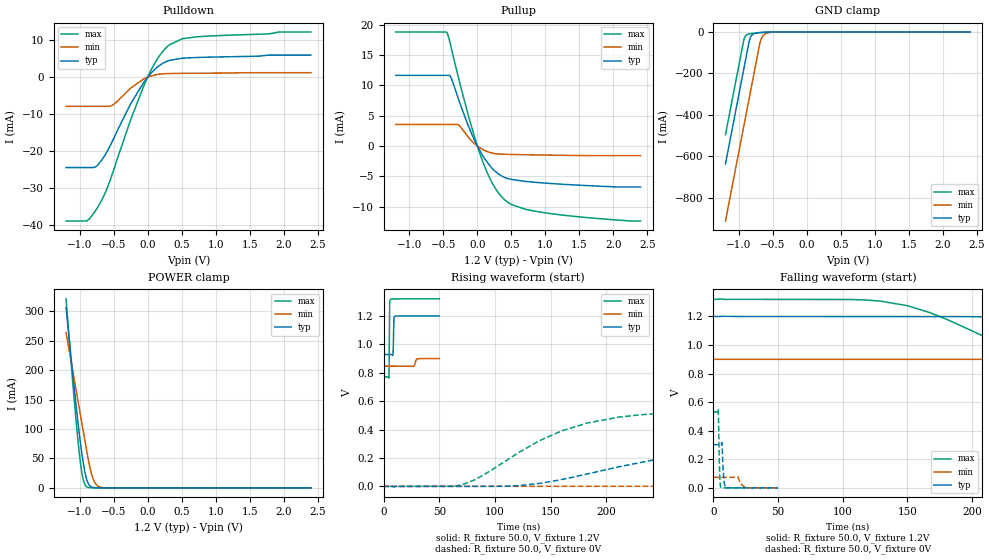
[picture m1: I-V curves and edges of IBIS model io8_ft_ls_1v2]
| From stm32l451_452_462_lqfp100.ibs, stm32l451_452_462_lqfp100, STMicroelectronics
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[Model]   io8_ft_ls_1v2
Model_type I/O
Polarity   Non-Inverting
Enable   Active-Low
| CAP_THRESHOLD on pad IOFT is "UDTCAPC" :
| Rising=30.00f vddiom   Falling=70.00f vddiom
| C_comp min and max val. don't necessarily correlate with the min and max pvt
| but are the smallest and greatest pad capacitance found.
| var   typ   min   max
C_comp   1.83455pF  1.76050pF  1.83491pF
|C_comp_pullup   1.06365pF  1.01770pF  1.04720pF
|C_comp_pulldown   770.90000fF  742.80001fF  787.71000fF
Vinl = 270.0mV
Vinh = 924.0mV
Vmeas = 600.0mV   | Reference voltage for timing measurements
Cref  = 50.0pF   | Timing specification test load capacitance value
Rref  = 100.0MOhm   | Timing specification test load resistance value
Vref  = 600.0mV   | Timing specification test load voltage
[Model Spec]
| TIME_THRESHOLD on pin ZIV12 is "CMOS" :
| Rising=50.00f vdd   Falling=50.00f vdd
Vinl 458.70000mV 364.70000mV 499.70000mV
Vinh 728.30000mV 548.30000mV 792.30000mV
| variable   typ   min   max
[Temperature Range] 25.0 140.0 -40.0
| variable   typ   min   max
[Voltage Range] 1.2V 900.0mV 1.32V
| variable   typ   min   max
[POWER Clamp Reference] 1.2V 900.0mV 1.32V
| variable   typ   min   max
[GND Clamp Reference] 0V 0V 0V
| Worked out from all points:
|   slope of the pulldown table from 0 to 0.18 V, typ, clamps not added: 55.6 ohm
|   slope of the pullup table from 0 to 0.18 V, typ, clamps not added: 56.3 ohm
|   GND clamp passes 1 mA (typ) near -0.61 V on its own axis
|   POWER clamp passes 1 mA (typ) near -0.81 V on its own axis
|   rising waveform, R_fixture 50.0, V_fixture 1.2V: 20-80 % time 432ps typ, 1.3ns min, 278ps max; typ from 0.928 V to 1.2 V
|   falling waveform, R_fixture 50.0, V_fixture 1.2V: 20-80 % time 167ns typ, 491ns min, 99.5ns max; typ from 1.2 V to 0.928 V
|   rising waveform, R_fixture 50.0, V_fixture 0V: 20-80 % time 127ns typ, 295ns min, 78.9ns max; typ from 0 V to 0.302 V
|   falling waveform, R_fixture 50.0, V_fixture 0V: 20-80 % time 1.14ns typ, 2.98ns min, 786ps max; typ from 0.302 V to 0 V
[POWER Clamp]
-1.2V     306.2mA    263.9mA    321.2mA
-1.09V    180mA      191mA      163.4mA
-1.05V    136.9mA    164.5mA    110.9mA
-1.01V    96.55mA    138mA      64.02mA
-960mV    52.29mA    104.9mA    20.68mA
-930mV    31.08mA    85.01mA    7.282mA
-900mV    15.67mA    65.13mA    2.025mA
-850mV    3.417mA    35.2mA     196.2uA
-800mV    570.2uA    14.97mA    18.13uA
-750mV    88.98uA    4.952mA    1.667uA
-680mV    6.495uA    823.9uA    58.96nA
2.4V      0A         0A         0A
[GND Clamp]
-1.2V     -636.9mA   -913.2mA   -495.8mA
-940mV    -194.9mA   -471.2mA   -53.78mA
-920mV    -160.9mA   -437.2mA   -28.06mA
-890mV    -109.9mA   -386.2mA   -14.28mA
-850mV    -43.09mA   -318.2mA   -9.18mA
-820mV    -18.33mA   -267.2mA   -7.516mA
-780mV    -7.695mA   -199.2mA   -5.87mA
-690mV    -2.548mA   -49.42mA   -2.9mA
-660mV    -1.868mA   -24.06mA   -2.112mA
-630mV    -1.326mA   -12.18mA   -1.447mA
-430mV    -19.32uA   -177.8uA   -8.091uA
2.4V      300pA      77.2nA     208.1pA
| variable   typ   min   max
[Pullup Reference] 1.2V 900.0mV 1.32V
| variable   typ   min   max
[Pulldown Reference] 0V 0V 0V
[Pullup]
-1.2V     11.66mA    3.558mA    18.8mA
-450mV    11.66mA    3.558mA    18.75mA
-390mV    11.34mA    3.558mA    16.48mA
-280mV    7.814mA    3.503mA    11.36mA
-110mV    2.689mA    1.153mA    4.138mA
50mV      -1.039mA   -379.5uA   -1.685mA
140mV     -2.617mA   -893.8uA   -4.276mA
240mV     -3.942mA   -1.22mA    -6.527mA
430mV     -5.313mA   -1.379mA   -9.149mA
700mV     -5.836mA   -1.444mA   -10.42mA
1.08V     -6.193mA   -1.513mA   -11.17mA
2.4V      -6.768mA   -1.592mA   -12.38mA
[Pulldown]
-1.2V     -24.47mA   -7.9mA     -38.94mA
-890mV    -24.47mA   -7.9mA     -38.83mA
-720mV    -23.49mA   -7.9mA     -34.76mA
-610mV    -20.54mA   -7.9mA     -30.69mA
-510mV    -17.01mA   -7.489mA   -25.69mA
-250mV    -7.205mA   -2.955mA   -11.53mA
0V        -16fA      0A         0A
160mV     2.97mA     779.8uA    5.417mA
320mV     4.547mA    983.4uA    8.763mA
510mV     5.135mA    1.031mA    10.4mA
700mV     5.311mA    1.057mA    10.88mA
2.4V      5.965mA    1.209mA    12.22mA
[Ramp]
dV/dt_r 181.26172mV/127.09367ns 44.06031mV/295.17618ns 319.20445mV/78.91734ns
dV/dt_f 162.93173mV/166.53891ns 32.17941mV/468.67509ns 329.57818mV/99.46975ns
R_load = 50.0
| Removed startup time: 0s 0s 0s  .
| Removed end time: 49.9ns.
[Rising Waveform]
R_fixture   = 50.0
V_fixture   = 1.2V
V_fixture_min = 900.0mV
V_fixture_max = 1.32V
0s        928.4mV    846.3mV    770.7mV
4.8ns     928.5mV    846.4mV    763.2mV
5.1ns     928.5mV    846.4mV    887.9mV
5.3ns     928.5mV    846.4mV    1.143V
5.5ns     928.5mV    846.4mV    1.284V
6.1ns     928.5mV    846.4mV    1.316V
8.4ns     926.5mV    846.4mV    1.32V
9.3ns     1.171V     846.4mV    1.32V
10.1ns    1.197V     846.4mV    1.32V
49.9ns    1.2V       899.9mV    1.32V
| Removed startup time: 0s 0s 0s  .
| Removed end time: 2.9999us.
[Falling Waveform]
R_fixture   = 50.0
V_fixture   = 1.2V
V_fixture_min = 900.0mV
V_fixture_max = 1.32V
0s        1.2V       900mV      1.32V
128.4ns   1.2V       900mV      1.309V
167.6ns   1.2V       900mV      1.227V
244ns     1.189V     900mV      938.9mV
267.2ns   1.176V     900mV      887.1mV
312.7ns   1.136V     900mV      829.5mV
416.9ns   1.017V     900mV      784.2mV
527.1ns   960.2mV    899.9mV    773.6mV
789.5ns   931.6mV    897.9mV    770.8mV
3us       928.4mV    846.4mV    770.7mV
| Removed startup time: 0s 0s 0s  .
| Removed end time: 1.9999us.
[Rising Waveform]
R_fixture   = 50.0
V_fixture   = 0V
V_fixture_min = 0V
V_fixture_max = 0V
0s        -21.55uV   -19.21uV   -16.72uV
70.8ns    -14.52uV   -5.362uV   12.13mV
121.2ns   5.11mV     -2.911uV   237.5mV
159.7ns   48.13mV    4.858uV    390.3mV
210.7ns   136.7mV    43.95uV    487mV
277.5ns   227.6mV    269.3uV    522.7mV
328.2ns   266.1mV    1.529mV    529.1mV
483.4ns   299.5mV    19.45mV    532mV
966.6ns   302.1mV    70.44mV    532mV
2us       302.1mV    73.43mV    532mV
| Removed startup time: 0s 0s 0s  .
| Removed end time: 49.9ns.
[Falling Waveform]
R_fixture   = 50.0
V_fixture   = 0V
V_fixture_min = 0V
V_fixture_max = 0V
0s        302.1mV    73.45mV    532mV
3.9ns     302.1mV    73.44mV    547.9mV
4.8ns     302mV      73.44mV    150.4mV
5.8ns     301.1mV    73.44mV    2.967mV
6.7ns     315mV      73.44mV    1.089mV
8.1ns     72.96mV    73.44mV    240.9uV
9.7ns     1.263mV    73.44mV    103.6uV
18.9ns    18.32uV    77.83mV    27.76uV
26.1ns    15.27uV    960.1uV    26.42uV
49.9ns    16.04uV    8.939uV    27.43uV
